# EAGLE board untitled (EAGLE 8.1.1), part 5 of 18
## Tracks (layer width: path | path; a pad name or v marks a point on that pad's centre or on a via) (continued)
S$4437 (continued)
  Bottom 0: 199.17,136.38 199.14,136.46
S$4438
  Bottom 0: 199.14,136.46 199.09,136.54
S$4439
  Bottom 0: 199.09,136.54 199.03,136.6
S$4440
  Bottom 0: 199.03,136.6 195.35,140.29
S$4441
  Bottom 0: 195.35,140.29 195.39,140.59
S$4442
  Bottom 0: 195.39,140.59 195.34,140.91
S$4443
  Bottom 0: 195.34,140.91 195.2,141.21
S$4444
  Bottom 0: 195.2,141.21 194.99,141.45
S$4445
  Bottom 0: 194.99,141.45 194.71,141.63
S$4446
  Bottom 0: 194.71,141.63 194.68,141.64
S$4447
  Bottom 0: 194.68,141.64 194.94,141.64
S$4448
  Bottom 0: 194.94,141.64 205.76,130.81
S$4449
  Bottom 0: 205.76,130.81 205.76,125.83
S$4450
  Bottom 0: 205.76,125.83 205.64,125.77
S$4451
  Bottom 0: 205.64,125.77 205.41,125.54
S$4452
  Bottom 0: 205.41,125.54 205.23,125.27
S$4453
  Bottom 0: 205.23,125.27 205.15,124.95
S$4454
  Bottom 0: 205.15,124.95 205.15,124.63
S$4455
  Bottom 0: 205.15,124.63 205.23,124.31
S$4456
  Bottom 0: 205.23,124.31 205.41,124.04
S$4457
  Bottom 0: 205.41,124.04 205.64,123.81
S$4458
  Bottom 0: 205.64,123.81 205.76,123.75
S$4459
  Bottom 0: 205.76,123.75 205.76,116.95
S$4460
  Bottom 0: 205.76,116.95 204.7,115.89
S$4461
  Bottom 0: 204.7,115.89 204.74,116.01
S$4462
  Bottom 0: 204.74,116.01 204.78,116.46
S$4463
  Bottom 0: 204.78,116.46 204.74,116.91
S$4464
  Bottom 0: 204.74,116.91 204.61,117.33
S$4465
  Bottom 0: 204.61,117.33 204.4,117.73
S$4466
  Bottom 0: 204.4,117.73 204.11,118.07
S$4467
  Bottom 0: 204.11,118.07 203.77,118.36
S$4468
  Bottom 0: 203.77,118.36 203.37,118.57
S$4469
  Bottom 0: 203.37,118.57 202.95,118.7
S$4470
  Bottom 0: 202.95,118.7 202.5,118.75
S$4471
  Bottom 0: 202.5,118.75 202.05,118.7
S$4472
  Bottom 0: 202.05,118.7 201.62,118.57
S$4473
  Bottom 0: 201.62,118.57 201.23,118.36
S$4474
  Bottom 0: 201.23,118.36 200.88,118.07
S$4475
  Bottom 0: 200.88,118.07 200.6,117.73
S$4476
  Bottom 0: 200.6,117.73 200.39,117.33
S$4477
  Bottom 0: 200.39,117.33 200.26,116.91
S$4478
  Bottom 0: 200.26,116.91 200.21,116.46
S$4479
  Bottom 0: 200.21,116.46 200.26,116.01
S$4480
  Bottom 0: 200.26,116.01 200.39,115.58
S$4481
  Bottom 0: 200.39,115.58 200.6,115.19
S$4482
  Bottom 0: 200.6,115.19 200.88,114.84
S$4483
  Bottom 0: 200.88,114.84 201.23,114.56
S$4484
  Bottom 0: 201.23,114.56 201.62,114.35
S$4485
  Bottom 0: 201.62,114.35 202.05,114.22
S$4486
  Bottom 0: 202.05,114.22 202.5,114.17
S$4487
  Bottom 0: 202.5,114.17 202.95,114.22
S$4488
  Bottom 0: 202.95,114.22 203.37,114.35
S$4489
  Bottom 0: 203.37,114.35 203.38,114.35
S$4490
  Bottom 0: 203.38,114.35 203.38,106.78
S$4491
  Bottom 0: 203.38,106.78 203.26,106.72
S$4492
  Bottom 0: 203.26,106.72 203.03,106.49
S$4493
  Bottom 0: 203.03,106.49 202.85,106.22
S$4494
  Bottom 0: 202.85,106.22 202.77,105.9
S$4495
  Bottom 0: 202.77,105.9 202.77,105.58
S$4496
  Bottom 0: 202.77,105.58 202.85,105.26
S$4497
  Bottom 0: 202.85,105.26 203.03,104.99
S$4498
  Bottom 0: 203.03,104.99 203.26,104.77
S$4499
  Bottom 0: 203.26,104.77 203.55,104.62
S$4500
  Bottom 0: 203.55,104.62 203.87,104.55
S$4501
  Bottom 0: 203.87,104.55 204.2,104.57
S$4502
  Bottom 0: 204.2,104.57 204.5,104.68
S$4503
  Bottom 0: 204.5,104.68 204.76,104.87
S$4504
  Bottom 0: 204.76,104.87 204.97,105.12
S$4505
  Bottom 0: 204.97,105.12 205.1,105.42
S$4506
  Bottom 0: 205.1,105.42 205.15,105.74
S$4507
  Bottom 0: 205.15,105.74 205.1,106.06
S$4508
  Bottom 0: 205.1,106.06 204.97,106.36
S$4509
  Bottom 0: 204.97,106.36 204.76,106.61
S$4510
  Bottom 0: 204.76,106.61 204.52,106.79
S$4511
  Bottom 0: 204.52,106.79 204.52,114.1
S$4512
  Bottom 0: 204.52,114.1 206.73,116.32
S$4513
  Bottom 0: 206.73,116.32 206.79,116.38
S$4514
  Bottom 0: 206.79,116.38 206.84,116.46
S$4515
  Bottom 0: 206.84,116.46 206.87,116.54
S$4516
  Bottom 0: 206.87,116.54 206.89,116.63
S$4517
  Bottom 0: 206.89,116.63 206.9,116.72
S$4518
  Bottom 0: 206.9,116.72 206.9,123.74
S$4519
  Bottom 0: 206.9,123.74 207.14,123.92
S$4520
  Bottom 0: 207.14,123.92 207.25,124.05
S$4521
  Bottom 0: 207.25,124.05 207.25,115.49
S$4522
  Bottom 0: 207.25,115.49 206.92,115.16
S$4523
  Bottom 0: 206.92,115.16 206.74,115.25
S$4524
  Bottom 0: 206.74,115.25 206.4,115.31
S$4525
  Bottom 0: 206.4,115.31 206.04,115.29
S$4526
  Bottom 0: 206.04,115.29 205.72,115.18
S$4527
  Bottom 0: 205.72,115.18 205.42,115
S$4528
  Bottom 0: 205.42,115 205.18,114.74
S$4529
  Bottom 0: 205.18,114.74 205.01,114.43
S$4530
  Bottom 0: 205.01,114.43 204.92,114.09
S$4531
  Bottom 0: 204.92,114.09 204.92,113.75
S$4532
  Bottom 0: 204.92,113.75 205.01,113.41
S$4533
  Bottom 0: 205.01,113.41 205.18,113.1
S$4534
  Bottom 0: 205.18,113.1 205.42,112.84
S$4535
  Bottom 0: 205.42,112.84 205.72,112.65
S$4536
  Bottom 0: 205.72,112.65 206.04,112.55
S$4537
  Bottom 0: 206.04,112.55 206.4,112.53
S$4538
  Bottom 0: 206.4,112.53 206.74,112.59
S$4539
  Bottom 0: 206.74,112.59 206.92,112.67
S$4540
  Bottom 0: 206.92,112.67 218.83,100.77
S$4541
  Bottom 0: 218.83,100.77 218.89,100.73
S$4542
  Bottom 0: 218.89,100.73 218.95,100.69
S$4543
  Bottom 0: 218.95,100.69 219.01,100.67
S$4544
  Bottom 0: 219.01,100.67 219.07,100.65
S$4545
  Bottom 0: 219.07,100.65 219.15,100.64
S$4546
  Bottom 0: 219.15,100.64 223.74,100.64
S$4547
  Bottom 0: 223.74,100.64 224.93,99.46
S$4548
  Bottom 0: 224.93,99.46 224.81,99.52
S$4549
  Bottom 0: 224.81,99.52 224.38,99.65
S$4550
  Bottom 0: 224.38,99.65 223.93,99.69
S$4551
  Bottom 0: 223.93,99.69 223.48,99.65
S$4552
  Bottom 0: 223.48,99.65 223.06,99.52
S$4553
  Bottom 0: 223.06,99.52 222.66,99.31
S$4554
  Bottom 0: 222.66,99.31 222.32,99.02
S$4555
  Bottom 0: 222.32,99.02 222.03,98.68
S$4556
  Bottom 0: 222.03,98.68 221.82,98.28
S$4557
  Bottom 0: 221.82,98.28 221.69,97.86
S$4558
  Bottom 0: 221.69,97.86 221.64,97.41
S$4559
  Bottom 0: 221.64,97.41 221.69,96.96
S$4560
  Bottom 0: 221.69,96.96 221.82,96.53
S$4561
  Bottom 0: 221.82,96.53 222.03,96.14
S$4562
  Bottom 0: 222.03,96.14 222.32,95.79
S$4563
  Bottom 0: 222.32,95.79 222.66,95.51
S$4564
  Bottom 0: 222.66,95.51 223.06,95.3
S$4565
  Bottom 0: 223.06,95.3 223.48,95.17
S$4566
  Bottom 0: 223.48,95.17 223.93,95.12
S$4567
  Bottom 0: 223.93,95.12 224.38,95.17
S$4568
  Bottom 0: 224.38,95.17 224.81,95.3
S$4569
  Bottom 0: 224.81,95.3 225.2,95.51
S$4570
  Bottom 0: 225.2,95.51 225.55,95.79
S$4571
  Bottom 0: 225.55,95.79 225.83,96.14
S$4572
  Bottom 0: 225.83,96.14 226.04,96.53
S$4573
  Bottom 0: 226.04,96.53 226.17,96.96
S$4574
  Bottom 0: 226.17,96.96 226.22,97.41
S$4575
  Bottom 0: 226.22,97.41 226.17,97.86
S$4576
  Bottom 0: 226.17,97.86 226.04,98.28
S$4577
  Bottom 0: 226.04,98.28 225.98,98.41
S$4578
  Bottom 0: 225.98,98.41 227.3,97.08
S$4579
  Bottom 0: 227.3,97.08 227.3,96.19
S$4580
  Bottom 0: 227.3,96.19 227.15,96.13
S$4581
  Bottom 0: 227.15,96.13 226.85,95.95
S$4582
  Bottom 0: 226.85,95.95 226.61,95.69
S$4583
  Bottom 0: 226.61,95.69 226.44,95.38
S$4584
  Bottom 0: 226.44,95.38 226.35,95.04
S$4585
  Bottom 0: 226.35,95.04 226.35,94.7
S$4586
  Bottom 0: 226.35,94.7 226.44,94.36
S$4587
  Bottom 0: 226.44,94.36 226.61,94.05
S$4588
  Bottom 0: 226.61,94.05 226.85,93.79
S$4589
  Bottom 0: 226.85,93.79 226.95,93.73
S$4590
  Bottom 0: 226.95,93.73 224.85,93.73
S$4591
  Bottom 0: 224.85,93.73 224.34,94.24
S$4592
  Bottom 0: 224.34,94.24 224.28,94.28
S$4593
  Bottom 0: 224.28,94.28 224.22,94.32
S$4594
  Bottom 0: 224.22,94.32 224.16,94.35
S$4595
  Bottom 0: 224.16,94.35 224.09,94.36
S$4596
  Bottom 0: 224.09,94.36 224.02,94.37
S$4597
  Bottom 0: 224.02,94.37 216.73,94.37
S$4598
  Bottom 0: 216.73,94.37 216.66,94.36
S$4599
  Bottom 0: 216.66,94.36 216.59,94.35
S$4600
  Bottom 0: 216.59,94.35 216.53,94.31
S$4601
  Bottom 0: 216.53,94.31 216.47,94.28
S$4602
  Bottom 0: 216.47,94.28 216.41,94.23
S$4603
  Bottom 0: 216.41,94.23 215.3,93.12
S$4604
  Bottom 0: 215.3,93.12 215.14,93.12
S$4605
  Bottom 0: 215.14,93.12 215.26,93.25
S$4606
  Bottom 0: 215.26,93.25 215.4,93.53
S$4607
  Bottom 0: 215.4,93.53 215.44,93.83
S$4608
  Bottom 0: 215.44,93.83 215.4,94.13
S$4609
  Bottom 0: 215.4,94.13 215.26,94.4
S$4610
  Bottom 0: 215.26,94.4 215.06,94.62
S$4611
  Bottom 0: 215.06,94.62 214.8,94.77
S$4612
  Bottom 0: 214.8,94.77 214.5,94.84
S$4613
  Bottom 0: 214.5,94.84 214.2,94.82
S$4614
  Bottom 0: 214.2,94.82 213.92,94.71
S$4615
  Bottom 0: 213.92,94.71 213.68,94.52
S$4616
  Bottom 0: 213.68,94.52 213.51,94.27
S$4617
  Bottom 0: 213.51,94.27 213.42,93.98
S$4618
  Bottom 0: 213.42,93.98 213.42,93.67
S$4619
  Bottom 0: 213.42,93.67 213.51,93.39
S$4620
  Bottom 0: 213.51,93.39 213.68,93.14
S$4621
  Bottom 0: 213.68,93.14 213.7,93.12
S$4622
  Bottom 0: 213.7,93.12 206.31,93.12
S$4623
  Bottom 0: 214.5,100.44 214.8,100.5
S$4624
  Bottom 0: 214.8,100.5 215.06,100.66
S$4625
  Bottom 0: 215.06,100.66 215.26,100.87
S$4626
  Bottom 0: 215.26,100.87 215.4,101.15
S$4627
  Bottom 0: 215.4,101.15 215.44,101.45
S$4628
  Bottom 0: 215.44,101.45 215.4,101.75
S$4629
  Bottom 0: 215.4,101.75 215.26,102.02
S$4630
  Bottom 0: 215.26,102.02 215.06,102.24
S$4631
  Bottom 0: 215.06,102.24 214.8,102.39
S$4632
  Bottom 0: 214.8,102.39 214.5,102.46
S$4633
  Bottom 0: 214.5,102.46 214.2,102.44
S$4634
  Bottom 0: 214.2,102.44 213.92,102.33
S$4635
  Bottom 0: 213.92,102.33 213.68,102.14
S$4636
  Bottom 0: 213.68,102.14 213.51,101.89
S$4637
  Bottom 0: 213.51,101.89 213.42,101.6
S$4638
  Bottom 0: 213.42,101.6 213.42,101.3
S$4639
  Bottom 0: 213.42,101.3 213.51,101.01
S$4640
  Bottom 0: 213.51,101.01 213.68,100.76
S$4641
  Bottom 0: 213.68,100.76 213.92,100.57
S$4642
  Bottom 0: 213.92,100.57 214.2,100.46
S$4643
  Bottom 0: 214.2,100.46 214.5,100.44
S$4644
  Bottom 0: 200.04,109.99 200.39,110.05
S$4645
  Bottom 0: 200.39,110.05 200.71,110.2
S$4646
  Bottom 0: 200.71,110.2 200.97,110.42
S$4647
  Bottom 0: 200.97,110.42 201.18,110.71
S$4648
  Bottom 0: 201.18,110.71 201.31,111.03
S$4649
  Bottom 0: 201.31,111.03 201.36,111.38
S$4650
  Bottom 0: 201.36,111.38 201.31,111.72
S$4651
  Bottom 0: 201.31,111.72 201.18,112.05
S$4652
  Bottom 0: 201.18,112.05 200.97,112.33
S$4653
  Bottom 0: 200.97,112.33 200.71,112.56
S$4654
  Bottom 0: 200.71,112.56 200.39,112.71
S$4655
  Bottom 0: 200.39,112.71 200.04,112.77
S$4656
  Bottom 0: 200.04,112.77 199.69,112.75
S$4657
  Bottom 0: 199.69,112.75 199.37,112.64
S$4658
  Bottom 0: 199.37,112.64 199.34,112.63
S$4659
  Bottom 0: 199.34,112.63 198.77,113.2
S$4660
  Bottom 0: 198.77,113.2 198.71,113.24
S$4661
  Bottom 0: 198.71,113.24 198.65,113.28
S$4662
  Bottom 0: 198.65,113.28 198.59,113.3
S$4663
  Bottom 0: 198.59,113.3 198.52,113.32
S$4664
  Bottom 0: 198.52,113.32 198.46,113.33
S$4665
  Bottom 0: 198.46,113.33 193.89,113.33
S$4666
  Bottom 0: 193.89,113.33 193.82,113.46
S$4667
  Bottom 0: 193.82,113.46 193.62,113.67
S$4668
  Bottom 0: 193.62,113.67 193.36,113.83
S$4669
  Bottom 0: 193.36,113.83 193.06,113.89
S$4670
  Bottom 0: 193.06,113.89 192.76,113.87
S$4671
  Bottom 0: 192.76,113.87 192.48,113.76
S$4672
  Bottom 0: 192.48,113.76 192.24,113.57
S$4673
  Bottom 0: 192.24,113.57 192.07,113.33
S$4674
  Bottom 0: 192.07,113.33 191.98,113.03
S$4675
  Bottom 0: 191.98,113.03 191.98,112.73
S$4676
  Bottom 0: 191.98,112.73 192.07,112.44
S$4677
  Bottom 0: 192.07,112.44 192.24,112.19
S$4678
  Bottom 0: 192.24,112.19 192.48,112
S$4679
  Bottom 0: 192.48,112 192.76,111.89
S$4680
  Bottom 0: 192.76,111.89 193.06,111.87
S$4681
  Bottom 0: 193.06,111.87 193.36,111.94
S$4682
  Bottom 0: 193.36,111.94 193.62,112.09
S$4683
  Bottom 0: 193.62,112.09 193.82,112.31
S$4684
  Bottom 0: 193.82,112.31 193.89,112.44
S$4685
  Bottom 0: 193.89,112.44 198.27,112.44
S$4686
  Bottom 0: 198.27,112.44 198.71,111.99
S$4687
  Bottom 0: 198.71,111.99 198.66,111.89
S$4688
  Bottom 0: 198.66,111.89 198.57,111.55
S$4689
  Bottom 0: 198.57,111.55 198.57,111.21
S$4690
  Bottom 0: 198.57,111.21 198.66,110.87
S$4691
  Bottom 0: 198.66,110.87 198.83,110.56
S$4692
  Bottom 0: 198.83,110.56 199.07,110.3
S$4693
  Bottom 0: 199.07,110.3 199.37,110.11
S$4694
  Bottom 0: 199.37,110.11 199.69,110.01
S$4695
  Bottom 0: 199.69,110.01 200.04,109.99
S$4696
  Bottom 0: 202.59,130.92 202.89,130.99
S$4697
  Bottom 0: 202.89,130.99 203.15,131.14
S$4698
  Bottom 0: 203.15,131.14 203.35,131.36
S$4699
  Bottom 0: 203.35,131.36 203.49,131.63
S$4700
  Bottom 0: 203.49,131.63 203.53,131.93
S$4701
  Bottom 0: 203.53,131.93 203.49,132.23
S$4702
  Bottom 0: 203.49,132.23 203.35,132.51
S$4703
  Bottom 0: 203.35,132.51 203.15,132.72
S$4704
  Bottom 0: 203.15,132.72 202.89,132.88
S$4705
  Bottom 0: 202.89,132.88 202.59,132.94
S$4706
  Bottom 0: 202.59,132.94 202.29,132.92
S$4707
  Bottom 0: 202.29,132.92 202.01,132.81
S$4708
  Bottom 0: 202.01,132.81 201.77,132.62
S$4709
  Bottom 0: 201.77,132.62 201.6,132.38
S$4710
  Bottom 0: 201.6,132.38 201.51,132.09
S$4711
  Bottom 0: 201.51,132.09 201.51,131.78
S$4712
  Bottom 0: 201.51,131.78 201.6,131.49
S$4713
  Bottom 0: 201.6,131.49 201.77,131.24
S$4714
  Bottom 0: 201.77,131.24 202.01,131.05
S$4715
  Bottom 0: 202.01,131.05 202.29,130.94
S$4716
  Bottom 0: 202.29,130.94 202.59,130.92
S$4717
  Bottom 0: 56.98,93.45 54.59,95.84
S$4718
  Bottom 0: 54.59,95.84 54.54,95.88
S$4719
  Bottom 0: 54.54,95.88 54.48,95.92
S$4720
  Bottom 0: 54.48,95.92 54.42,95.95
S$4721
  Bottom 0: 54.42,95.95 54.35,95.96
S$4722
  Bottom 0: 54.35,95.96 54.28,95.97
S$4723
  Bottom 0: 54.28,95.97 38.09,95.97
S$4724
  Bottom 0: 38.09,95.97 37.99,96.05
S$4725
  Bottom 0: 37.99,96.05 37.67,96.2
S$4726
  Bottom 0: 37.67,96.2 37.33,96.26
S$4727
  Bottom 0: 37.33,96.26 36.98,96.24
S$4728
  Bottom 0: 36.98,96.24 36.65,96.13
S$4729
  Bottom 0: 36.65,96.13 36.35,95.95
S$4730
  Bottom 0: 36.35,95.95 36.11,95.69
S$4731
  Bottom 0: 36.11,95.69 35.94,95.38
S$4732
  Bottom 0: 35.94,95.38 35.92,95.31
S$4733
  Bottom 0: 35.92,95.31 34.34,95.31
S$4734
  Bottom 0: 34.34,95.31 34.7,95.51
S$4735
  Bottom 0: 34.7,95.51 35.05,95.79
S$4736
  Bottom 0: 35.05,95.79 35.33,96.14
S$4737
  Bottom 0: 35.33,96.14 35.55,96.53
S$4738
  Bottom 0: 35.55,96.53 35.67,96.96
S$4739
  Bottom 0: 35.67,96.96 35.72,97.41
S$4740
  Bottom 0: 35.72,97.41 35.67,97.86
S$4741
  Bottom 0: 35.67,97.86 35.55,98.28
S$4742
  Bottom 0: 35.55,98.28 35.33,98.68
S$4743
  Bottom 0: 35.33,98.68 35.05,99.02
S$4744
  Bottom 0: 35.05,99.02 34.7,99.31
S$4745
  Bottom 0: 34.7,99.31 34.3,99.52
S$4746
  Bottom 0: 34.3,99.52
S$4747
  Bottom 0: 34.3,99.52 34.34,99.55
S$4748
  Bottom 0: 34.34,99.55 34.39,99.59
S$4749
  Bottom 0: 34.39,99.59 36.89,102.08
S$4750
  Bottom 0: 36.89,102.08 40.97,102.08
S$4751
  Bottom 0: 40.97,102.08 40.85,101.97
S$4752
  Bottom 0: 40.85,101.97 40.67,101.69
S$4753
  Bottom 0: 40.67,101.69 40.59,101.38
S$4754
  Bottom 0: 40.59,101.38 40.59,101.05
S$4755
  Bottom 0: 40.59,101.05 40.67,100.74
S$4756
  Bottom 0: 40.67,100.74 40.85,100.46
S$4757
  Bottom 0: 40.85,100.46 41.08,100.24
S$4758
  Bottom 0: 41.08,100.24 41.37,100.09
S$4759
  Bottom 0: 41.37,100.09 41.69,100.03
S$4760
  Bottom 0: 41.69,100.03 42.01,100.05
S$4761
  Bottom 0: 42.01,100.05 42.11,100.08
S$4762
  Bottom 0: 42.11,100.08 42.43,99.75
S$4763
  Bottom 0: 42.43,99.75 42.5,99.69
S$4764
  Bottom 0: 42.5,99.69 42.58,99.64
S$4765
  Bottom 0: 42.58,99.64 42.66,99.61
S$4766
  Bottom 0: 42.66,99.61 42.74,99.59
S$4767
  Bottom 0: 42.74,99.59 42.84,99.58
S$4768
  Bottom 0: 42.84,99.58 56.58,99.58
S$4769
  Bottom 0: 56.58,99.58 56.37,99.52
S$4770
  Bottom 0: 56.37,99.52 55.98,99.31
S$4771
  Bottom 0: 55.98,99.31 55.63,99.02
S$4772
  Bottom 0: 55.63,99.02 55.34,98.68
S$4773
  Bottom 0: 55.34,98.68 55.13,98.28
S$4774
  Bottom 0: 55.13,98.28 55,97.86
S$4775
  Bottom 0: 55,97.86 54.96,97.41
S$4776
  Bottom 0: 54.96,97.41 55,96.96
S$4777
  Bottom 0: 55,96.96 55.13,96.53
S$4778
  Bottom 0: 55.13,96.53 55.34,96.14
S$4779
  Bottom 0: 55.34,96.14 55.63,95.79
S$4780
  Bottom 0: 55.63,95.79 55.98,95.51
S$4781
  Bottom 0: 55.98,95.51 56.37,95.3
S$4782
  Bottom 0: 56.37,95.3 56.8,95.17
S$4783
  Bottom 0: 56.8,95.17 57.25,95.12
S$4784
  Bottom 0: 57.25,95.12 57.69,95.17
S$4785
  Bottom 0: 57.69,95.17 58.12,95.3
S$4786
  Bottom 0: 58.12,95.3 58.52,95.51
S$4787
  Bottom 0: 58.52,95.51 58.86,95.79
S$4788
  Bottom 0: 58.86,95.79 59.15,96.14
S$4789
  Bottom 0: 59.15,96.14 59.36,96.53
S$4790
  Bottom 0: 59.36,96.53 59.49,96.96
S$4791
  Bottom 0: 59.49,96.96 59.53,97.41
S$4792
  Bottom 0: 59.53,97.41 59.49,97.86
S$4793
  Bottom 0: 59.49,97.86 59.36,98.28
S$4794
  Bottom 0: 59.36,98.28 59.15,98.68
S$4795
  Bottom 0: 59.15,98.68 58.86,99.02
S$4796
  Bottom 0: 58.86,99.02 58.52,99.31
S$4797
  Bottom 0: 58.52,99.31 58.12,99.52
S$4798
  Bottom 0: 58.12,99.52 57.92,99.58
S$4799
  Bottom 0: 57.92,99.58 58.23,99.58
S$4800
  Bottom 0: 58.23,99.58 58.33,99.59
S$4801
  Bottom 0: 58.33,99.59 58.41,99.61
S$4802
  Bottom 0: 58.41,99.61 58.49,99.64
S$4803
  Bottom 0: 58.49,99.64 58.57,99.69
S$4804
  Bottom 0: 58.57,99.69 58.64,99.75
S$4805
  Bottom 0: 58.64,99.75 61.46,102.57
S$4806
  Bottom 0: 61.46,102.57 61.52,102.64
S$4807
  Bottom 0: 61.52,102.64 61.57,102.71
S$4808
  Bottom 0: 61.57,102.71 61.6,102.79
S$4809
  Bottom 0: 61.6,102.79 61.62,102.88
S$4810
  Bottom 0: 61.62,102.88 61.63,102.97
S$4811
  Bottom 0: 61.63,102.97 61.63,104.69
S$4812
  Bottom 0: 61.63,104.69 61.87,104.87
S$4813
  Bottom 0: 61.87,104.87 62.08,105.12
S$4814
  Bottom 0: 62.08,105.12 62.21,105.42
S$4815
  Bottom 0: 62.21,105.42 62.26,105.74
S$4816
  Bottom 0: 62.26,105.74 62.21,106.06
S$4817
  Bottom 0: 62.21,106.06 62.08,106.36
S$4818
  Bottom 0: 62.08,106.36 61.87,106.61
S$4819
  Bottom 0: 61.87,106.61 61.61,106.8
S$4820
  Bottom 0: 61.61,106.8 61.3,106.91
S$4821
  Bottom 0: 61.3,106.91 60.98,106.93
S$4822
  Bottom 0: 60.98,106.93 60.73,106.88
S$4823
  Bottom 0: 60.73,106.88 58.74,108.86
S$4824
  Bottom 0: 58.74,108.86 58.74,112.39
S$4825
  Bottom 0: 58.74,112.39 58.88,112.19
S$4826
  Bottom 0: 58.88,112.19 59.12,112
S$4827
  Bottom 0: 59.12,112 59.4,111.89
S$4828
  Bottom 0: 59.4,111.89 59.7,111.87
S$4829
  Bottom 0: 59.7,111.87 59.99,111.94
S$4830
  Bottom 0: 59.99,111.94 60.26,112.09
S$4831
  Bottom 0: 60.26,112.09 60.46,112.31
S$4832
  Bottom 0: 60.46,112.31 60.53,112.44
S$4833
  Bottom 0: 60.53,112.44 64.92,112.44
S$4834
  Bottom 0: 64.92,112.44 65.36,111.99
S$4835
  Bottom 0: 65.36,111.99 65.31,111.89
S$4836
  Bottom 0: 65.31,111.89 65.22,111.55
S$4837
  Bottom 0: 65.22,111.55 65.22,111.21
S$4838
  Bottom 0: 65.22,111.21 65.31,110.87
S$4839
  Bottom 0: 65.31,110.87 65.48,110.56
S$4840
  Bottom 0: 65.48,110.56 65.72,110.3
S$4841
  Bottom 0: 65.72,110.3 66.01,110.11
S$4842
  Bottom 0: 66.01,110.11 66.34,110.01
S$4843
  Bottom 0: 66.34,110.01 66.69,109.99
S$4844
  Bottom 0: 66.69,109.99 67.04,110.05
S$4845
  Bottom 0: 67.04,110.05 67.35,110.2
S$4846
  Bottom 0: 67.35,110.2 67.62,110.42
S$4847
  Bottom 0: 67.62,110.42 67.83,110.71
S$4848
  Bottom 0: 67.83,110.71 67.96,111.03
S$4849
  Bottom 0: 67.96,111.03 68.01,111.38
S$4850
  Bottom 0: 68.01,111.38 67.96,111.72
S$4851
  Bottom 0: 67.96,111.72 67.83,112.05
S$4852
  Bottom 0: 67.83,112.05 67.62,112.33
S$4853
  Bottom 0: 67.62,112.33 67.35,112.56
S$4854
  Bottom 0: 67.35,112.56 67.04,112.71
S$4855
  Bottom 0: 67.04,112.71 66.69,112.77
S$4856
  Bottom 0: 66.69,112.77 66.34,112.75
S$4857
  Bottom 0: 66.34,112.75 66.01,112.64
S$4858
  Bottom 0: 66.01,112.64 65.99,112.63
S$4859
  Bottom 0: 65.99,112.63 65.42,113.2
S$4860
  Bottom 0: 65.42,113.2 65.36,113.24
S$4861
  Bottom 0: 65.36,113.24 65.3,113.28
S$4862
  Bottom 0: 65.3,113.28 65.24,113.3
S$4863
  Bottom 0: 65.24,113.3 65.18,113.32
S$4864
  Bottom 0: 65.18,113.32 65.11,113.33
S$4865
  Bottom 0: 65.11,113.33 60.53,113.33
S$4866
  Bottom 0: 60.53,113.33 60.46,113.46
S$4867
  Bottom 0: 60.46,113.46 60.26,113.67
S$4868
  Bottom 0: 60.26,113.67 59.99,113.83
S$4869
  Bottom 0: 59.99,113.83 59.7,113.89
S$4870
  Bottom 0: 59.7,113.89 59.4,113.87
S$4871
  Bottom 0: 59.4,113.87 59.12,113.76
S$4872
  Bottom 0: 59.12,113.76 58.88,113.57
S$4873
  Bottom 0: 58.88,113.57 58.74,113.37
S$4874
  Bottom 0: 58.74,113.37 58.74,120.02
S$4875
  Bottom 0: 58.74,120.02 58.88,119.81
S$4876
  Bottom 0: 58.88,119.81 59.12,119.62
S$4877
  Bottom 0: 59.12,119.62 59.4,119.51
S$4878
  Bottom 0: 59.4,119.51 59.7,119.49
S$4879
  Bottom 0: 59.7,119.49 59.99,119.56
S$4880
  Bottom 0: 59.99,119.56 60.26,119.71
S$4881
  Bottom 0: 60.26,119.71 60.46,119.93
S$4882
  Bottom 0: 60.46,119.93 60.59,120.2
S$4883
  Bottom 0: 60.59,120.2 60.64,120.5
S$4884
  Bottom 0: 60.64,120.5 60.59,120.8
S$4885
  Bottom 0: 60.59,120.8 60.46,121.08
S$4886
  Bottom 0: 60.46,121.08 60.26,121.3
S$4887
  Bottom 0: 60.26,121.3 59.99,121.45
S$4888
  Bottom 0: 59.99,121.45 59.7,121.51
S$4889
  Bottom 0: 59.7,121.51 59.4,121.49
S$4890
  Bottom 0: 59.4,121.49 59.12,121.38
S$4891
  Bottom 0: 59.12,121.38 58.88,121.19
S$4892
  Bottom 0: 58.88,121.19 58.71,120.94
S$4893
  Bottom 0: 58.71,120.94 58.67,120.81
S$4894
  Bottom 0: 58.67,120.81 58.63,120.87
S$4895
  Bottom 0: 58.63,120.87 58.57,120.93
S$4896
  Bottom 0: 58.57,120.93 55.06,124.45
S$4897
  Bottom 0: 55.06,124.45 55.06,124.47
S$4898
  Bottom 0: 55.06,124.47 55.11,124.79
S$4899
  Bottom 0: 55.11,124.79 55.06,125.11
S$4900
  Bottom 0: 55.06,125.11 54.93,125.41
S$4901
  Bottom 0: 54.93,125.41 54.73,125.66
S$4902
  Bottom 0: 54.73,125.66 54.46,125.85
S$4903
  Bottom 0: 54.46,125.85 54.26,125.92
S$4904
  Bottom 0: 54.26,125.92 65,125.92
S$4905
  Bottom 0: 65,125.92 64.95,125.91
S$4906
  Bottom 0: 64.95,125.91 64.66,125.77
S$4907
  Bottom 0: 64.66,125.77 64.42,125.54
S$4908
  Bottom 0: 64.42,125.54 64.25,125.27
S$4909
  Bottom 0: 64.25,125.27 64.17,124.95
S$4910
  Bottom 0: 64.17,124.95 64.17,124.63
S$4911
  Bottom 0: 64.17,124.63 64.25,124.31
S$4912
  Bottom 0: 64.25,124.31 64.42,124.04
S$4913
  Bottom 0: 64.42,124.04 64.66,123.81
S$4914
  Bottom 0: 64.66,123.81 64.95,123.67
S$4915
  Bottom 0: 64.95,123.67 65.27,123.6
S$4916
  Bottom 0: 65.27,123.6 65.59,123.62
S$4917
  Bottom 0: 65.59,123.62 65.81,123.7
S$4918
  Bottom 0: 65.81,123.7 66.86,122.65
S$4919
  Bottom 0: 66.86,122.65 66.84,122.63
S$4920
  Bottom 0: 66.84,122.63 66.79,122.58
S$4921
  Bottom 0: 66.79,122.58 66.74,122.5
S$4922
  Bottom 0: 66.74,122.5 66.74,122.43
S$4923
  Bottom 0: 66.74,122.43 66.74,120.65
S$4924
  Bottom 0: 66.74,120.65 66.74,120.57
S$4925
  Bottom 0: 66.74,120.57 66.79,120.5
S$4926
  Bottom 0: 66.79,120.5 66.84,120.45
S$4927
  Bottom 0: 66.84,120.45 66.91,120.41
S$4928
  Bottom 0: 66.91,120.41 66.99,120.4
S$4929
  Bottom 0: 66.99,120.4 68.77,120.4
S$4930
  Bottom 0: 68.77,120.4 68.82,120.4
S$4931
  Bottom 0: 68.82,120.4 71.17,118.05
S$4932
  Bottom 0: 71.17,118.05 71.17,117.5
S$4933
  Bottom 0: 71.17,117.5 71.05,117.73
S$4934
  Bottom 0: 71.05,117.73 70.76,118.07
S$4935
  Bottom 0: 70.76,118.07 70.42,118.36
S$4936
  Bottom 0: 70.42,118.36 70.02,118.57
S$4937
  Bottom 0: 70.02,118.57 69.6,118.7
S$4938
  Bottom 0: 69.6,118.7 69.15,118.75
S$4939
  Bottom 0: 69.15,118.75 68.7,118.7
S$4940
  Bottom 0: 68.7,118.7 68.27,118.57
S$4941
  Bottom 0: 68.27,118.57 67.88,118.36
S$4942
  Bottom 0: 67.88,118.36 67.53,118.07
S$4943
  Bottom 0: 67.53,118.07 67.25,117.73
S$4944
  Bottom 0: 67.25,117.73 67.03,117.33
S$4945
  Bottom 0: 67.03,117.33 66.91,116.91
S$4946
  Bottom 0: 66.91,116.91 66.86,116.46
S$4947
  Bottom 0: 66.86,116.46 66.91,116.01
S$4948
  Bottom 0: 66.91,116.01 67.03,115.58
S$4949
  Bottom 0: 67.03,115.58 67.25,115.19
S$4950
  Bottom 0: 67.25,115.19 67.53,114.84
S$4951
  Bottom 0: 67.53,114.84 67.88,114.56
S$4952
  Bottom 0: 67.88,114.56 68.27,114.35
S$4953
  Bottom 0: 68.27,114.35 68.7,114.22
S$4954
  Bottom 0: 68.7,114.22 69.15,114.17
S$4955
  Bottom 0: 69.15,114.17 69.6,114.22
S$4956
  Bottom 0: 69.6,114.22 69.91,114.31
S$4957
  Bottom 0: 69.91,114.31
S$4958
  Bottom 0: 69.91,114.31 69.87,114.25
S$4959
  Bottom 0: 69.87,114.25 69.84,114.19
S$4960
  Bottom 0: 69.84,114.19 69.83,114.12
S$4961
  Bottom 0: 69.83,114.12 69.82,114.05
S$4962
  Bottom 0: 69.82,114.05 69.82,109.13
S$4963
  Bottom 0: 69.82,109.13 69.68,108.98
S$4964
  Bottom 0: 69.68,108.98 69.59,108.74
S$4965
  Bottom 0: 69.59,108.74 69.59,108.49
S$4966
  Bottom 0: 69.59,108.49 69.68,108.25
S$4967
  Bottom 0: 69.68,108.25 69.82,108.1
S$4968
  Bottom 0: 69.82,108.1 69.82,104.27
S$4969
  Bottom 0: 69.82,104.27 61.67,96.11
S$4970
  Bottom 0: 61.67,96.11 61.49,96.2
S$4971
  Bottom 0: 61.49,96.2 61.14,96.26
S$4972
  Bottom 0: 61.14,96.26 60.79,96.24
S$4973
  Bottom 0: 60.79,96.24 60.46,96.13
S$4974
  Bottom 0: 60.46,96.13 60.17,95.95
S$4975
  Bottom 0: 60.17,95.95 59.93,95.69
S$4976
  Bottom 0: 59.93,95.69 59.76,95.38
S$4977
  Bottom 0: 59.76,95.38 59.67,95.04
S$4978
  Bottom 0: 59.67,95.04 59.67,94.7
S$4979
  Bottom 0: 59.67,94.7 59.76,94.36
S$4980
  Bottom 0: 59.76,94.36 59.93,94.05
S$4981
  Bottom 0: 59.93,94.05 60.17,93.79
S$4982
  Bottom 0: 60.17,93.79 60.46,93.6
S$4983
  Bottom 0: 60.46,93.6 60.79,93.5
S$4984
  Bottom 0: 60.79,93.5 61.14,93.48
S$4985
  Bottom 0: 61.14,93.48 61.49,93.54
S$4986
  Bottom 0: 61.49,93.54 61.8,93.69
S$4987
  Bottom 0: 61.8,93.69 62.07,93.91
S$4988
  Bottom 0: 62.07,93.91 62.28,94.2
S$4989
  Bottom 0: 62.28,94.2 62.41,94.52
S$4990
  Bottom 0: 62.41,94.52 62.45,94.87
S$4991
  Bottom 0: 62.45,94.87 62.41,95.21
S$4992
  Bottom 0: 62.41,95.21 62.3,95.48
S$4993
  Bottom 0: 62.3,95.48 70.58,103.77
S$4994
  Bottom 0: 70.58,103.77 70.62,103.83
S$4995
  Bottom 0: 70.62,103.83 70.66,103.89
S$4996
  Bottom 0: 70.66,103.89 70.69,103.95
S$4997
  Bottom 0: 70.69,103.95 70.7,104.01
S$4998
  Bottom 0: 70.7,104.01 70.71,104.08
S$4999
  Bottom 0: 70.71,104.08 70.71,108.1
S$5000
  Bottom 0: 70.71,108.1 70.78,108.15
S$5001
  Bottom 0: 70.78,108.15 70.9,108.37
S$5002
  Bottom 0: 70.9,108.37 70.95,108.61
S$5003
  Bottom 0: 70.95,108.61 70.9,108.86
S$5004
  Bottom 0: 70.9,108.86 70.78,109.08
S$5005
  Bottom 0: 70.78,109.08 70.71,109.13
S$5006
  Bottom 0: 70.71,109.13 70.71,113.86
S$5007
  Bottom 0: 70.71,113.86 71.92,115.08
S$5008
  Bottom 0: 71.92,115.08 71.97,115.14
S$5009
  Bottom 0: 71.97,115.14 72.01,115.2
S$5010
  Bottom 0: 72.01,115.2 72.03,115.26
S$5011
  Bottom 0: 72.03,115.26 72.05,115.33
S$5012
  Bottom 0: 72.05,115.33 72.05,115.4
S$5013
  Bottom 0: 72.05,115.4 72.05,118.24
S$5014
  Bottom 0: 72.05,118.24 72.05,118.31
S$5015
  Bottom 0: 72.05,118.31 72.03,118.37
S$5016
  Bottom 0: 72.03,118.37 72.01,118.44
S$5017
  Bottom 0: 72.01,118.44 71.97,118.5
S$5018
  Bottom 0: 71.97,118.5 71.92,118.55
S$5019
  Bottom 0: 71.92,118.55 70,120.48
S$5020
  Bottom 0: 70,120.48 70.26,120.41
S$5021
  Bottom 0: 70.26,120.41 70.58,120.41
S$5022
  Bottom 0: 70.58,120.41 70.71,120.45
S$5023
  Bottom 0: 70.71,120.45 75.35,115.81
S$5024
  Bottom 0: 75.35,115.81 75.35,113.13
S$5025
  Bottom 0: 75.35,113.13 75.35,113.04
S$5026
  Bottom 0: 75.35,113.04 75.37,112.95
S$5027
  Bottom 0: 75.37,112.95 75.41,112.87
S$5028
  Bottom 0: 75.41,112.87 75.45,112.8
S$5029
  Bottom 0: 75.45,112.8 75.51,112.73
S$5030
  Bottom 0: 75.51,112.73 90.62,97.62
S$5031
  Bottom 0: 90.62,97.62 90.58,97.44
S$5032
  Bottom 0: 90.58,97.44 90.58,97.12
S$5033
  Bottom 0: 90.58,97.12 90.67,96.8
S$5034
  Bottom 0: 90.67,96.8 90.84,96.53
S$5035
  Bottom 0: 90.84,96.53 91.07,96.31
S$5036
  Bottom 0: 91.07,96.31 91.36,96.16
S$5037
  Bottom 0: 91.36,96.16 91.68,96.09
S$5038
  Bottom 0: 91.68,96.09 92.01,96.11
S$5039
  Bottom 0: 92.01,96.11 92.31,96.22
S$5040
  Bottom 0: 92.31,96.22 92.58,96.41
S$5041
  Bottom 0: 92.58,96.41 92.78,96.66
S$5042
  Bottom 0: 92.78,96.66 92.91,96.96
S$5043
  Bottom 0: 92.91,96.96 92.96,97.28
S$5044
  Bottom 0: 92.96,97.28 92.91,97.6
S$5045
  Bottom 0: 92.91,97.6 92.78,97.9
S$5046
  Bottom 0: 92.78,97.9 92.58,98.16
S$5047
  Bottom 0: 92.58,98.16 92.31,98.34
S$5048
  Bottom 0: 92.31,98.34 92.01,98.45
S$5049
  Bottom 0: 92.01,98.45 91.68,98.47
S$5050
  Bottom 0: 91.68,98.47 91.43,98.42
S$5051
  Bottom 0: 91.43,98.42 76.49,113.36
S$5052
  Bottom 0: 76.49,113.36 76.69,113.26
S$5053
  Bottom 0: 76.69,113.26 76.93,113.24
S$5054
  Bottom 0: 76.93,113.24 77.18,113.3
S$5055
  Bottom 0: 77.18,113.3 77.38,113.46
S$5056
  Bottom 0: 77.38,113.46 77.51,113.67
S$5057
  Bottom 0: 77.51,113.67 77.56,113.92
S$5058
  Bottom 0: 77.56,113.92 77.51,114.17
S$5059
  Bottom 0: 77.51,114.17 77.38,114.38
S$5060
  Bottom 0: 77.38,114.38 77.31,114.43
S$5061
  Bottom 0: 77.31,114.43 77.31,122.48
S$5062
  Bottom 0: 77.31,122.48 85.42,130.59
S$5063
  Bottom 0: 85.42,130.59 85.47,130.64
S$5064
  Bottom 0: 85.47,130.64 85.51,130.7
S$5065
  Bottom 0: 85.51,130.7 85.53,130.76
S$5066
  Bottom 0: 85.53,130.76 85.55,130.83
S$5067
  Bottom 0: 85.55,130.83 85.55,130.9
S$5068
  Bottom 0: 85.55,130.9 85.55,151.58
S$5069
  Bottom 0: 85.55,151.58 95.45,151.58
S$5070
  Bottom 0: 95.45,151.58 95.47,151.51
S$5071
  Bottom 0: 95.47,151.51 95.64,151.2
S$5072
  Bottom 0: 95.64,151.2 95.89,150.94
S$5073
  Bottom 0: 95.89,150.94 96.18,150.75
S$5074
  Bottom 0: 96.18,150.75 96.51,150.65
S$5075
  Bottom 0: 96.51,150.65 96.86,150.63
S$5076
  Bottom 0: 96.86,150.63 97.21,150.69
S$5077
  Bottom 0: 97.21,150.69 97.52,150.84
S$5078
  Bottom 0: 97.52,150.84 97.79,151.06
S$5079
  Bottom 0: 97.79,151.06 98,151.35
S$5080
  Bottom 0: 98,151.35 98.12,151.67
S$5081
  Bottom 0: 98.12,151.67 98.17,152.02
S$5082
  Bottom 0: 98.17,152.02 98.12,152.36
S$5083
  Bottom 0: 98.12,152.36 98,152.69
S$5084
  Bottom 0: 98,152.69 97.79,152.97
S$5085
  Bottom 0: 97.79,152.97 97.52,153.2
S$5086
  Bottom 0: 97.52,153.2 97.21,153.35
S$5087
  Bottom 0: 97.21,153.35 96.86,153.41
S$5088
  Bottom 0: 96.86,153.41 96.51,153.39
S$5089
  Bottom 0: 96.51,153.39 96.18,153.28
S$5090
  Bottom 0: 96.18,153.28 95.89,153.1
S$5091
  Bottom 0: 95.89,153.1 95.64,152.84
S$5092
  Bottom 0: 95.64,152.84 95.47,152.53
S$5093
  Bottom 0: 95.47,152.53 95.45,152.46
S$5094
  Bottom 0: 95.45,152.46 93.87,152.46
S$5095
  Bottom 0: 93.87,152.46 94.23,152.66
S$5096
  Bottom 0: 94.23,152.66 94.58,152.94
S$5097
  Bottom 0: 94.58,152.94 94.86,153.29
S$5098
  Bottom 0: 94.86,153.29 95.08,153.68
S$5099
  Bottom 0: 95.08,153.68 95.2,154.11
S$5100
  Bottom 0: 95.2,154.11 95.25,154.56
S$5101
  Bottom 0: 95.25,154.56 95.2,155.01
S$5102
  Bottom 0: 95.2,155.01 95.08,155.43
S$5103
  Bottom 0: 95.08,155.43 94.86,155.83
S$5104
  Bottom 0: 94.86,155.83 94.58,156.17
S$5105
  Bottom 0: 94.58,156.17 94.23,156.46
S$5106
  Bottom 0: 94.23,156.46 93.84,156.67
S$5107
  Bottom 0: 93.84,156.67 93.41,156.8
S$5108
  Bottom 0: 93.41,156.8 92.96,156.84
S$5109
  Bottom 0: 92.96,156.84 92.52,156.8
S$5110
  Bottom 0: 92.52,156.8 92.09,156.67
S$5111
  Bottom 0: 92.09,156.67 91.69,156.46
S$5112
  Bottom 0: 91.69,156.46 91.35,156.17
S$5113
  Bottom 0: 91.35,156.17 91.06,155.83
S$5114
  Bottom 0: 91.06,155.83 90.85,155.43
S$5115
  Bottom 0: 90.85,155.43 90.72,155.01
S$5116
  Bottom 0: 90.72,155.01 90.68,154.56
S$5117
  Bottom 0: 90.68,154.56 90.72,154.11
S$5118
  Bottom 0: 90.72,154.11 90.85,153.68
S$5119
  Bottom 0: 90.85,153.68 91.06,153.29
S$5120
  Bottom 0: 91.06,153.29 91.35,152.94
S$5121
  Bottom 0: 91.35,152.94 91.69,152.66
S$5122
  Bottom 0: 91.69,152.66 92.06,152.46
S$5123
  Bottom 0: 92.06,152.46 85.3,152.46
S$5124
  Bottom 0: 85.3,152.46 74.8,162.96
S$5125
  Bottom 0: 74.8,162.96 74.8,164.2
S$5126
  Bottom 0: 74.8,164.2 74.87,164.25
S$5127
  Bottom 0: 74.87,164.25 75,164.46
S$5128
  Bottom 0: 75,164.46 75.05,164.71
S$5129
  Bottom 0: 75.05,164.71 75.03,164.79
S$5130
  Bottom 0: 75.03,164.79 76.59,163.23
S$5131
  Bottom 0: 76.59,163.23 76.55,163.06
S$5132
  Bottom 0: 76.55,163.06 76.55,162.73
S$5133
  Bottom 0: 76.55,162.73 76.63,162.42
S$5134
  Bottom 0: 76.63,162.42 76.81,162.14
S$5135
  Bottom 0: 76.81,162.14 77.04,161.92
S$5136
  Bottom 0: 77.04,161.92 77.33,161.77
S$5137
  Bottom 0: 77.33,161.77 77.65,161.71
S$5138
  Bottom 0: 77.65,161.71 77.97,161.73
S$5139
  Bottom 0: 77.97,161.73 78.28,161.83
S$5140
  Bottom 0: 78.28,161.83 78.54,162.02
S$5141
  Bottom 0: 78.54,162.02 78.75,162.28
S$5142
  Bottom 0: 78.75,162.28 78.77,162.33
S$5143
  Bottom 0: 78.77,162.33 84.88,162.33
S$5144
  Bottom 0: 84.88,162.33 84.97,162.33
S$5145
  Bottom 0: 84.97,162.33 85.06,162.35
S$5146
  Bottom 0: 85.06,162.35 85.14,162.38
S$5147
  Bottom 0: 85.14,162.38 85.22,162.43
S$5148
  Bottom 0: 85.22,162.43 85.28,162.49
S$5149
  Bottom 0: 85.28,162.49 86.92,164.13
S$5150
  Bottom 0: 86.92,164.13 87.18,164.08
S$5151
  Bottom 0: 87.18,164.08 87.5,164.1
S$5152
  Bottom 0: 87.5,164.1 87.81,164.21
S$5153
  Bottom 0: 87.81,164.21 88.07,164.4
S$5154
  Bottom 0: 88.07,164.4 88.28,164.65
S$5155
  Bottom 0: 88.28,164.65 88.3,164.7
S$5156
  Bottom 0: 88.3,164.7 94.17,164.7
S$5157
  Bottom 0: 94.17,164.7 95.64,163.23
S$5158
  Bottom 0: 95.64,163.23 95.6,163.06
S$5159
  Bottom 0: 95.6,163.06 95.6,162.73
S$5160
  Bottom 0: 95.6,162.73 95.69,162.42
S$5161
  Bottom 0: 95.69,162.42 95.86,162.14
S$5162
  Bottom 0: 95.86,162.14 96.09,161.92
S$5163
  Bottom 0: 96.09,161.92 96.38,161.77
S$5164
  Bottom 0: 96.38,161.77 96.7,161.71
S$5165
  Bottom 0: 96.7,161.71 97.03,161.73
S$5166
  Bottom 0: 97.03,161.73 97.33,161.83
S$5167
  Bottom 0: 97.33,161.83 97.6,162.02
S$5168
  Bottom 0: 97.6,162.02 97.8,162.28
S$5169
  Bottom 0: 97.8,162.28 97.83,162.33
S$5170
  Bottom 0: 97.83,162.33 103.2,162.33
S$5171
  Bottom 0: 103.2,162.33 103.2,159.31
S$5172
  Bottom 0: 103.2,159.31 103.13,159.4
S$5173
  Bottom 0: 103.13,159.4 102.86,159.55
S$5174
  Bottom 0: 102.86,159.55 102.57,159.61
S$5175
  Bottom 0: 102.57,159.61 102.27,159.59
S$5176
  Bottom 0: 102.27,159.59 101.99,159.48
S$5177
  Bottom 0: 101.99,159.48 101.75,159.29
S$5178
  Bottom 0: 101.75,159.29 101.58,159.04
S$5179
  Bottom 0: 101.58,159.04 101.49,158.75
S$5180
  Bottom 0: 101.49,158.75 101.49,158.6
S$5181
  Bottom 0: 101.49,158.6 94.72,158.6
S$5182
  Bottom 0: 94.72,158.6 94.98,158.78
S$5183
  Bottom 0: 94.98,158.78 95.19,159.02
S$5184
  Bottom 0: 95.19,159.02 95.33,159.32
S$5185
  Bottom 0: 95.33,159.32 95.38,159.64
S$5186
  Bottom 0: 95.38,159.64 95.33,159.96
S$5187
  Bottom 0: 95.33,159.96 95.19,160.26
S$5188
  Bottom 0: 95.19,160.26 94.98,160.5
S$5189
  Bottom 0: 94.98,160.5 94.71,160.68
S$5190
  Bottom 0: 94.71,160.68 94.4,160.77
S$5191
  Bottom 0: 94.4,160.77 94.07,160.77
S$5192
  Bottom 0: 94.07,160.77 93.76,160.68
S$5193
  Bottom 0: 93.76,160.68 93.48,160.5
S$5194
  Bottom 0: 93.48,160.5 93.27,160.26
S$5195
  Bottom 0: 93.27,160.26 93.13,159.96
S$5196
  Bottom 0: 93.13,159.96 93.09,159.64
S$5197
  Bottom 0: 93.09,159.64 93.13,159.32
S$5198
  Bottom 0: 93.13,159.32 93.27,159.02
S$5199
  Bottom 0: 93.27,159.02 93.48,158.78
S$5200
  Bottom 0: 93.48,158.78 93.75,158.6
S$5201
  Bottom 0: 93.75,158.6 92.78,158.6
S$5202
  Bottom 0: 92.78,158.6 92.83,158.67
S$5203
  Bottom 0: 92.83,158.67 92.84,158.75
S$5204
  Bottom 0: 92.84,158.75 92.84,160.53
S$5205
  Bottom 0: 92.84,160.53 92.83,160.6
S$5206
  Bottom 0: 92.83,160.6 92.78,160.68
S$5207
  Bottom 0: 92.78,160.68 92.73,160.73
S$5208
  Bottom 0: 92.73,160.73 92.66,160.77
S$5209
  Bottom 0: 92.66,160.77 92.58,160.78
S$5210
  Bottom 0: 92.58,160.78 92.14,160.78
S$5211
  Bottom 0: 92.14,160.78 92.14,160.91
S$5212
  Bottom 0: 92.14,160.91 92.08,161.13
S$5213
  Bottom 0: 92.08,161.13 91.91,161.29
S$5214
  Bottom 0: 91.91,161.29 91.69,161.35
S$5215
  Bottom 0: 91.69,161.35 91.34,161.35
S$5216
  Bottom 0: 91.34,161.35 90.25,162.44
S$5217
  Bottom 0: 90.25,162.44 90.31,162.57
S$5218
  Bottom 0: 90.31,162.57 90.36,162.89
S$5219
  Bottom 0: 90.36,162.89 90.31,163.22
S$5220
  Bottom 0: 90.31,163.22 90.18,163.51
S$5221
  Bottom 0: 90.18,163.51 89.98,163.77
S$5222
  Bottom 0: 89.98,163.77 89.71,163.96
S$5223
  Bottom 0: 89.71,163.96 89.41,164.06
S$5224
  Bottom 0: 89.41,164.06 89.08,164.08
S$5225
  Bottom 0: 89.08,164.08 88.76,164.02
S$5226
  Bottom 0: 88.76,164.02 88.47,163.87
S$5227
  Bottom 0: 88.47,163.87 88.24,163.65
S$5228
  Bottom 0: 88.24,163.65 88.07,163.37
S$5229
  Bottom 0: 88.07,163.37 87.98,163.06
S$5230
  Bottom 0: 87.98,163.06 87.98,162.73
S$5231
  Bottom 0: 87.98,162.73 88.07,162.42
S$5232
  Bottom 0: 88.07,162.42 88.24,162.14
S$5233
  Bottom 0: 88.24,162.14 88.47,161.92
S$5234
  Bottom 0: 88.47,161.92 88.76,161.77
S$5235
  Bottom 0: 88.76,161.77 89.08,161.71
S$5236
  Bottom 0: 89.08,161.71 89.41,161.73
S$5237
  Bottom 0: 89.41,161.73 89.63,161.8
S$5238
  Bottom 0: 89.63,161.8 90.68,160.75
S$5239
  Bottom 0: 90.68,160.75 90.66,160.73
S$5240
  Bottom 0: 90.66,160.73 90.6,160.68
S$5241
  Bottom 0: 90.6,160.68 90.56,160.6
S$5242
  Bottom 0: 90.56,160.6 90.55,160.53
S$5243
  Bottom 0: 90.55,160.53 90.55,158.75
S$5244
  Bottom 0: 90.55,158.75 90.56,158.67
S$5245
  Bottom 0: 90.56,158.67 90.6,158.6
S$5246
  Bottom 0: 90.6,158.6 84.46,158.6
S$5247
  Bottom 0: 84.46,158.6 84.41,158.9
S$5248
  Bottom 0: 84.41,158.9 84.28,159.18
S$5249
  Bottom 0: 84.28,159.18 84.08,159.4
S$5250
  Bottom 0: 84.08,159.4 83.81,159.55
S$5251
  Bottom 0: 83.81,159.55 83.52,159.61
S$5252
  Bottom 0: 83.52,159.61 83.22,159.59
S$5253
  Bottom 0: 83.22,159.59 82.94,159.48
S$5254
  Bottom 0: 82.94,159.48 82.7,159.29
S$5255
  Bottom 0: 82.7,159.29 82.53,159.04
S$5256
  Bottom 0: 82.53,159.04 82.44,158.75
S$5257
  Bottom 0: 82.44,158.75 82.44,158.45
S$5258
  Bottom 0: 82.44,158.45 82.53,158.16
S$5259
  Bottom 0: 82.53,158.16 82.7,157.91
S$5260
  Bottom 0: 82.7,157.91 82.94,157.72
S$5261
  Bottom 0: 82.94,157.72 83.22,157.61
S$5262
  Bottom 0: 83.22,157.61 83.52,157.59
S$5263
  Bottom 0: 83.52,157.59 83.81,157.66
S$5264
  Bottom 0: 83.81,157.66 83.92,157.72
S$5265
  Bottom 0: 83.92,157.72 101.99,157.72
S$5266
  Bottom 0: 101.99,157.72 102.27,157.61
S$5267
  Bottom 0: 102.27,157.61 102.57,157.59
S$5268
  Bottom 0: 102.57,157.59 102.86,157.66
S$5269
  Bottom 0: 102.86,157.66 103.13,157.81
S$5270
  Bottom 0: 103.13,157.81 103.2,157.89
S$5271
  Bottom 0: 103.2,157.89 103.2,151.69
S$5272
  Bottom 0: 103.2,151.69 103.13,151.78
S$5273
  Bottom 0: 103.13,151.78 102.86,151.93
S$5274
  Bottom 0: 102.86,151.93 102.57,151.99
S$5275
  Bottom 0: 102.57,151.99 102.27,151.97
S$5276
  Bottom 0: 102.27,151.97 101.99,151.86
S$5277
  Bottom 0: 101.99,151.86 101.75,151.67
S$5278
  Bottom 0: 101.75,151.67 101.58,151.43
S$5279
  Bottom 0: 101.58,151.43 101.49,151.13
S$5280
  Bottom 0: 101.49,151.13 101.49,150.83
S$5281
  Bottom 0: 101.49,150.83 101.58,150.54
S$5282
  Bottom 0: 101.58,150.54 101.75,150.29
S$5283
  Bottom 0: 101.75,150.29 101.99,150.1
S$5284
  Bottom 0: 101.99,150.1 102.27,149.99
S$5285
  Bottom 0: 102.27,149.99 102.57,149.97
S$5286
  Bottom 0: 102.57,149.97 102.86,150.04
S$5287
  Bottom 0: 102.86,150.04 103.13,150.19
S$5288
  Bottom 0: 103.13,150.19 103.2,150.27
S$5289
  Bottom 0: 103.2,150.27 103.2,146.3
S$5290
  Bottom 0: 103.2,146.3 101.88,144.98
S$5291
  Bottom 0: 101.88,144.98 101.79,145.01
S$5292
  Bottom 0: 101.79,145.01 101.46,145.03
S$5293
  Bottom 0: 101.46,145.03 101.14,144.96
S$5294
  Bottom 0: 101.14,144.96 100.85,144.82
S$5295
  Bottom 0: 100.85,144.82 100.62,144.59
S$5296
  Bottom 0: 100.62,144.59 100.45,144.32
S$5297
  Bottom 0: 100.45,144.32 100.36,144
S$5298
  Bottom 0: 100.36,144 100.36,143.68
S$5299
  Bottom 0: 100.36,143.68 100.45,143.36
S$5300
  Bottom 0: 100.45,143.36 100.62,143.09
S$5301
  Bottom 0: 100.62,143.09 100.85,142.87
S$5302
  Bottom 0: 100.85,142.87 101.14,142.72
S$5303
  Bottom 0: 101.14,142.72 101.46,142.65
S$5304
  Bottom 0: 101.46,142.65 101.79,142.67
S$5305
  Bottom 0: 101.79,142.67 101.88,142.7
S$5306
  Bottom 0: 101.88,142.7 102.61,141.98
S$5307
  Bottom 0: 102.61,141.98 102.61,133.85
S$5308
  Bottom 0: 102.61,133.85 102.55,133.92
S$5309
  Bottom 0: 102.55,133.92 102.28,134.15
S$5310
  Bottom 0: 102.28,134.15 101.98,134.29
S$5311
  Bottom 0: 101.98,134.29 101.98,139.84
S$5312
  Bottom 0: 101.98,139.84 101.97,139.91
S$5313
  Bottom 0: 101.97,139.91 101.96,139.97
S$5314
  Bottom 0: 101.96,139.97 101.93,140.03
S$5315
  Bottom 0: 101.93,140.03 101.89,140.09
S$5316
  Bottom 0: 101.89,140.09 101.85,140.15
S$5317
  Bottom 0: 101.85,140.15 94.96,147.04
S$5318
  Bottom 0: 94.96,147.04 94.91,147.08
S$5319
  Bottom 0: 94.91,147.08 94.84,147.12
S$5320
  Bottom 0: 94.84,147.12 94.78,147.15
S$5321
  Bottom 0: 94.78,147.15 94.72,147.16
S$5322
  Bottom 0: 94.72,147.16 94.64,147.17
S$5323
  Bottom 0: 94.64,147.17 90.18,147.17
S$5324
  Bottom 0: 90.18,147.17 87.75,149.61
S$5325
  Bottom 0: 87.75,149.61 87.76,149.66
S$5326
  Bottom 0: 87.76,149.66 87.72,149.91
S$5327
  Bottom 0: 87.72,149.91 87.58,150.12
S$5328
  Bottom 0: 87.58,150.12 87.38,150.27
S$5329
  Bottom 0: 87.38,150.27 87.14,150.34
S$5330
  Bottom 0: 87.14,150.34 86.89,150.31
S$5331
  Bottom 0: 86.89,150.31 86.67,150.21
S$5332
  Bottom 0: 86.67,150.21 86.49,150.02
S$5333
  Bottom 0: 86.49,150.02 86.4,149.78
S$5334
  Bottom 0: 86.4,149.78 86.4,149.53
S$5335
  Bottom 0: 86.4,149.53 86.49,149.3
S$5336
  Bottom 0: 86.49,149.3 86.67,149.11
S$5337
  Bottom 0: 86.67,149.11 86.89,149
S$5338
  Bottom 0: 86.89,149 87.13,148.98
S$5339
  Bottom 0: 87.13,148.98 89.69,146.42
S$5340
  Bottom 0: 89.69,146.42 89.74,146.37
S$5341
  Bottom 0: 89.74,146.37 89.8,146.33
S$5342
  Bottom 0: 89.8,146.33 89.86,146.3
S$5343
  Bottom 0: 89.86,146.3 89.93,146.29
S$5344
  Bottom 0: 89.93,146.29 90,146.28
S$5345
  Bottom 0: 90,146.28 94.46,146.28
S$5346
  Bottom 0: 94.46,146.28 99.02,141.72
S$5347
  Bottom 0: 99.02,141.72 98.83,141.72
S$5348
  Bottom 0: 98.83,141.72 98.52,141.63
S$5349
  Bottom 0: 98.52,141.63 98.25,141.45
S$5350
  Bottom 0: 98.25,141.45 98.03,141.21
S$5351
  Bottom 0: 98.03,141.21 97.89,140.91
S$5352
  Bottom 0: 97.89,140.91 97.85,140.59
S$5353
  Bottom 0: 97.85,140.59 97.89,140.29
S$5354
  Bottom 0: 97.89,140.29 97.6,140
S$5355
  Bottom 0: 97.6,140 97.6,141.48
S$5356
  Bottom 0: 97.6,141.48 97.59,141.55
S$5357
  Bottom 0: 97.59,141.55 97.55,141.62
S$5358
  Bottom 0: 97.55,141.62 97.49,141.68
S$5359
  Bottom 0: 97.49,141.68 97.42,141.72
S$5360
  Bottom 0: 97.42,141.72 97.34,141.73
S$5361
  Bottom 0: 97.34,141.73 96.9,141.73
S$5362
  Bottom 0: 96.9,141.73 96.9,141.86
S$5363
  Bottom 0: 96.9,141.86 96.83,142.08
S$5364
  Bottom 0: 96.83,142.08 96.67,142.24
S$5365
  Bottom 0: 96.67,142.24 96.45,142.3
S$5366
  Bottom 0: 96.45,142.3 96.09,142.3
S$5367
  Bottom 0: 96.09,142.3 95.01,143.38
S$5368
  Bottom 0: 95.01,143.38 95.07,143.52
S$5369
  Bottom 0: 95.07,143.52 95.12,143.84
S$5370
  Bottom 0: 95.12,143.84 95.07,144.16
S$5371
  Bottom 0: 95.07,144.16 94.94,144.46
S$5372
  Bottom 0: 94.94,144.46 94.74,144.71
S$5373
  Bottom 0: 94.74,144.71 94.47,144.9
S$5374
  Bottom 0: 94.47,144.9 94.17,145.01
S$5375
  Bottom 0: 94.17,145.01 93.84,145.03
S$5376
  Bottom 0: 93.84,145.03 93.52,144.96
S$5377
  Bottom 0: 93.52,144.96 93.23,144.82
S$5378
  Bottom 0: 93.23,144.82 93,144.59
S$5379
  Bottom 0: 93,144.59 92.83,144.32
S$5380
  Bottom 0: 92.83,144.32 92.74,144
S$5381
  Bottom 0: 92.74,144 92.74,143.68
S$5382
  Bottom 0: 92.74,143.68 92.83,143.36
S$5383
  Bottom 0: 92.83,143.36 93,143.09
S$5384
  Bottom 0: 93,143.09 93.23,142.87
S$5385
  Bottom 0: 93.23,142.87 93.52,142.72
S$5386
  Bottom 0: 93.52,142.72 93.84,142.65
S$5387
  Bottom 0: 93.84,142.65 94.17,142.67
S$5388
  Bottom 0: 94.17,142.67 94.39,142.75
S$5389
  Bottom 0: 94.39,142.75 95.44,141.7
S$5390
  Bottom 0: 95.44,141.7 95.42,141.68
S$5391
  Bottom 0: 95.42,141.68 95.36,141.62
S$5392
  Bottom 0: 95.36,141.62 95.32,141.55
S$5393
  Bottom 0: 95.32,141.55 95.31,141.48
S$5394
  Bottom 0: 95.31,141.48 95.31,139.7
S$5395
  Bottom 0: 95.31,139.7 95.32,139.62
S$5396
  Bottom 0: 95.32,139.62 95.36,139.55
S$5397
  Bottom 0: 95.36,139.55 95.42,139.5
S$5398
  Bottom 0: 95.42,139.5 95.49,139.46
S$5399
  Bottom 0: 95.49,139.46 95.56,139.45
S$5400
  Bottom 0: 95.56,139.45 97.05,139.45
S$5401
  Bottom 0: 97.05,139.45 91.08,133.48
S$5402
  Bottom 0: 91.08,133.48 87,137.56
S$5403
  Bottom 0: 87,137.56 87,138.72
S$5404
  Bottom 0: 87,138.72 87.07,138.83
S$5405
  Bottom 0: 87.07,138.83 87.11,139.08
S$5406
  Bottom 0: 87.11,139.08 87.07,139.33
S$5407
  Bottom 0: 87.07,139.33 86.93,139.54
S$5408
  Bottom 0: 86.93,139.54 86.73,139.69
S$5409
  Bottom 0: 86.73,139.69 86.49,139.76
S$5410
  Bottom 0: 86.49,139.76 86.24,139.74
S$5411
  Bottom 0: 86.24,139.74 86.02,139.63
S$5412
  Bottom 0: 86.02,139.63 85.84,139.44
S$5413
  Bottom 0: 85.84,139.44 85.75,139.21
S$5414
  Bottom 0: 85.75,139.21 85.75,138.95
S$5415
  Bottom 0: 85.75,138.95 85.84,138.72
S$5416
  Bottom 0: 85.84,138.72 85.86,138.7
S$5417
  Bottom 0: 85.86,138.7 85.86,137.33
S$5418
  Bottom 0: 85.86,137.33 85.86,137.23
S$5419
  Bottom 0: 85.86,137.23 85.88,137.15
S$5420
  Bottom 0: 85.88,137.15 85.92,137.07
S$5421
  Bottom 0: 85.92,137.07 85.96,136.99
S$5422
  Bottom 0: 85.96,136.99 86.02,136.92
S$5423
  Bottom 0: 86.02,136.92 90.19,132.76
S$5424
  Bottom 0: 90.19,132.76 89.2,131.77
S$5425
  Bottom 0: 89.2,131.77 89.22,131.93
S$5426
  Bottom 0: 89.22,131.93 89.18,132.23
S$5427
  Bottom 0: 89.18,132.23 89.05,132.51
S$5428
  Bottom 0: 89.05,132.51 88.84,132.72
S$5429
  Bottom 0: 88.84,132.72 88.58,132.88
S$5430
  Bottom 0: 88.58,132.88 88.28,132.94
S$5431
  Bottom 0: 88.28,132.94 87.98,132.92
S$5432
  Bottom 0: 87.98,132.92 87.7,132.81
S$5433
  Bottom 0: 87.7,132.81 87.46,132.62
S$5434
  Bottom 0: 87.46,132.62 87.29,132.38
S$5435
  Bottom 0: 87.29,132.38 87.2,132.09
S$5436
  Bottom 0: 87.2,132.09 87.2,131.78
S$5437
  Bottom 0: 87.2,131.78 87.29,131.49
S$5438
  Bottom 0: 87.29,131.49 87.46,131.24
S$5439
  Bottom 0: 87.46,131.24 87.7,131.05
S$5440
  Bottom 0: 87.7,131.05 87.98,130.94
S$5441
  Bottom 0: 87.98,130.94 88.28,130.92
S$5442
  Bottom 0: 88.28,130.92 88.58,130.99
S$5443
  Bottom 0: 88.58,130.99 88.84,131.14
S$5444
  Bottom 0: 88.84,131.14 88.9,131.2
S$5445
  Bottom 0: 88.9,131.2 88.9,122.52
S$5446
  Bottom 0: 88.9,122.52 88.72,122.4
S$5447
  Bottom 0: 88.72,122.4 88.51,122.16
S$5448
  Bottom 0: 88.51,122.16 88.37,121.86
S$5449
  Bottom 0: 88.37,121.86 88.33,121.54
S$5450
  Bottom 0: 88.33,121.54 88.37,121.22
S$5451
  Bottom 0: 88.37,121.22 88.51,120.92
S$5452
  Bottom 0: 88.51,120.92 88.72,120.67
S$5453
  Bottom 0: 88.72,120.67 88.85,120.59
S$5454
  Bottom 0: 88.85,120.59 88.06,120.59
S$5455
  Bottom 0: 88.06,120.59 88.07,120.65
S$5456
  Bottom 0: 88.07,120.65 88.07,122.43
S$5457
  Bottom 0: 88.07,122.43 88.06,122.5
S$5458
  Bottom 0: 88.06,122.5 88.02,122.58
S$5459
  Bottom 0: 88.02,122.58 87.97,122.63
S$5460
  Bottom 0: 87.97,122.63 87.89,122.67
S$5461
  Bottom 0: 87.89,122.67 87.82,122.68
S$5462
  Bottom 0: 87.82,122.68 87.37,122.68
S$5463
  Bottom 0: 87.37,122.68 87.37,122.81
S$5464
  Bottom 0: 87.37,122.81 87.31,123.03
S$5465
  Bottom 0: 87.31,123.03 87.15,123.19
S$5466
  Bottom 0: 87.15,123.19 86.93,123.25
S$5467
  Bottom 0: 86.93,123.25 86.57,123.25
S$5468
  Bottom 0: 86.57,123.25 85.48,124.33
S$5469
  Bottom 0: 85.48,124.33 85.55,124.47
S$5470
  Bottom 0: 85.55,124.47 85.59,124.79
S$5471
  Bottom 0: 85.59,124.79 85.55,125.11
S$5472
  Bottom 0: 85.55,125.11 85.42,125.41
S$5473
  Bottom 0: 85.42,125.41 85.21,125.66
S$5474
  Bottom 0: 85.21,125.66 84.95,125.85
S$5475
  Bottom 0: 84.95,125.85 84.64,125.96
S$5476
  Bottom 0: 84.64,125.96 84.32,125.98
S$5477
  Bottom 0: 84.32,125.98 84,125.91
S$5478
  Bottom 0: 84,125.91 83.71,125.77
S$5479
  Bottom 0: 83.71,125.77 83.47,125.54
S$5480
  Bottom 0: 83.47,125.54 83.3,125.27
S$5481
  Bottom 0: 83.3,125.27 83.22,124.95
S$5482
  Bottom 0: 83.22,124.95 83.22,124.63
S$5483
  Bottom 0: 83.22,124.63 83.3,124.31
S$5484
  Bottom 0: 83.3,124.31 83.47,124.04
S$5485
  Bottom 0: 83.47,124.04 83.71,123.81
S$5486
  Bottom 0: 83.71,123.81 84,123.67
S$5487
  Bottom 0: 84,123.67 84.32,123.6
S$5488
  Bottom 0: 84.32,123.6 84.64,123.62
S$5489
  Bottom 0: 84.64,123.62 84.87,123.7
S$5490
  Bottom 0: 84.87,123.7 85.92,122.65
S$5491
  Bottom 0: 85.92,122.65 85.89,122.63
S$5492
  Bottom 0: 85.89,122.63 85.84,122.58
S$5493
  Bottom 0: 85.84,122.58 85.8,122.5
S$5494
  Bottom 0: 85.8,122.5 85.79,122.43
S$5495
  Bottom 0: 85.79,122.43 85.79,120.65
S$5496
  Bottom 0: 85.79,120.65 85.8,120.59
S$5497
  Bottom 0: 85.8,120.59 79.68,120.59
S$5498
  Bottom 0: 79.68,120.59 79.65,120.8
S$5499
  Bottom 0: 79.65,120.8 79.52,121.08
S$5500
  Bottom 0: 79.52,121.08 79.31,121.3
S$5501
  Bottom 0: 79.31,121.3 79.05,121.45
S$5502
  Bottom 0: 79.05,121.45 78.75,121.51
S$5503
  Bottom 0: 78.75,121.51 78.45,121.49
S$5504
  Bottom 0: 78.45,121.49 78.17,121.38
S$5505
  Bottom 0: 78.17,121.38 77.93,121.19
S$5506
  Bottom 0: 77.93,121.19 77.76,120.94
S$5507
  Bottom 0: 77.76,120.94 77.67,120.66
S$5508
  Bottom 0: 77.67,120.66 77.67,120.35
S$5509
  Bottom 0: 77.67,120.35 77.76,120.06
S$5510
  Bottom 0: 77.76,120.06 77.93,119.81
S$5511
  Bottom 0: 77.93,119.81 78.17,119.62
S$5512
  Bottom 0: 78.17,119.62 78.45,119.51
S$5513
  Bottom 0: 78.45,119.51 78.75,119.49
S$5514
  Bottom 0: 78.75,119.49 79.05,119.56
S$5515
  Bottom 0: 79.05,119.56 79.3,119.7
S$5516
  Bottom 0: 79.3,119.7 97.12,119.7
S$5517
  Bottom 0: 97.12,119.7 97.23,119.62
S$5518
  Bottom 0: 97.23,119.62 97.51,119.51
S$5519
  Bottom 0: 97.51,119.51 97.81,119.49
S$5520
  Bottom 0: 97.81,119.49 98.11,119.56
S$5521
  Bottom 0: 98.11,119.56 98.37,119.71
S$5522
  Bottom 0: 98.37,119.71 98.57,119.93
S$5523
  Bottom 0: 98.57,119.93 98.7,120.2
S$5524
  Bottom 0: 98.7,120.2 98.75,120.46
S$5525
  Bottom 0: 98.75,120.46 106.59,112.62
S$5526
  Bottom 0: 106.59,112.62 106.59,98.44
S$5527
  Bottom 0: 106.59,98.44 106.53,98.45
S$5528
  Bottom 0: 106.53,98.45 106.21,98.48
S$5529
  Bottom 0: 106.21,98.48 105.89,98.41
S$5530
  Bottom 0: 105.89,98.41 105.6,98.26
S$5531
  Bottom 0: 105.6,98.26 105.36,98.04
S$5532
  Bottom 0: 105.36,98.04 105.19,97.77
S$5533
  Bottom 0: 105.19,97.77 105.1,97.45
S$5534
  Bottom 0: 105.1,97.45 105.1,97.12
S$5535
  Bottom 0: 105.1,97.12 105.19,96.81
S$5536
  Bottom 0: 105.19,96.81 105.36,96.53
S$5537
  Bottom 0: 105.36,96.53 105.6,96.31
S$5538
  Bottom 0: 105.6,96.31 105.89,96.16
S$5539
  Bottom 0: 105.89,96.16 106.21,96.1
S$5540
  Bottom 0: 106.21,96.1 106.45,96.11
S$5541
  Bottom 0: 106.45,96.11 104.83,94.49
S$5542
  Bottom 0: 104.83,94.49 104.59,94.47
S$5543
  Bottom 0: 104.59,94.47 104.36,94.36
S$5544
  Bottom 0: 104.36,94.36 104.19,94.17
S$5545
  Bottom 0: 104.19,94.17 104.1,93.93
S$5546
  Bottom 0: 104.1,93.93 104.1,93.68
S$5547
